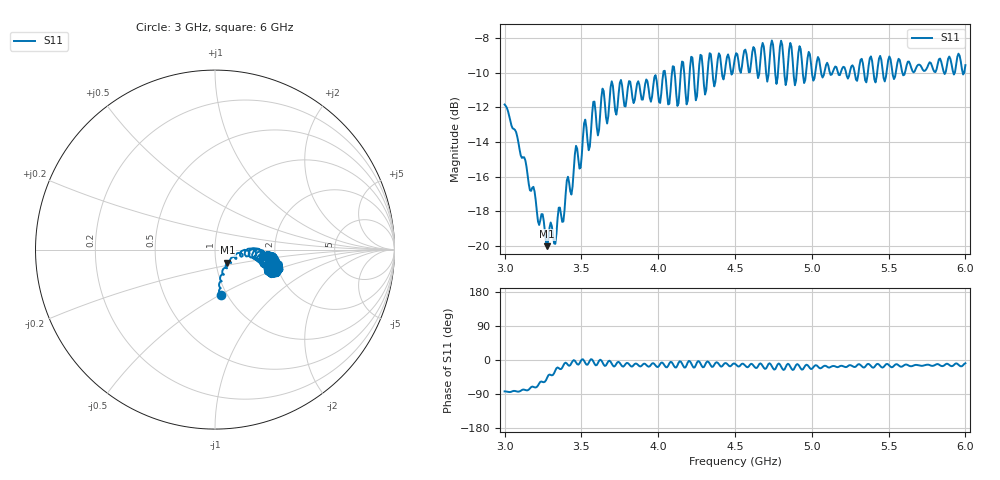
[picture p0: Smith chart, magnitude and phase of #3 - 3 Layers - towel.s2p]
!  02/07/2025  16:57:06
! Ref Plane: 0.000 mm
# MHZ S MA R  50
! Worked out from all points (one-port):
!   401 points, 3 GHz to 6 GHz, reference 50 ohm
!   lowest |S11| = -20.0 dB at 3.277 GHz (marker M1), VSWR 1.22, Z = 56.8 - j8.26 ohm
!   |S11| at or under -10 dB: start of sweep to 4.034 GHz; 4.044 GHz to 4.09 GHz (45.36 MHz wide, 1.12 % of centre); 4.107 GHz to 4.147 GHz (40.1 MHz wide, 0.972 % of centre)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
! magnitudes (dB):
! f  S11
! 3 GHz  -11.8
! 3.277 GHz  -20.0
! 3.375 GHz  -18.6
! 3.465 GHz  -14.2
! 3.555 GHz  -14.3
! 3.578 GHz  -11.7
! 3.607 GHz  -13.6
! 3.638 GHz  -10.9
! 3.667 GHz  -12.9
! 3.75 GHz  -10.6
! 4.013 GHz  -11.7
! 4.043 GHz  -9.9
! 4.065 GHz  -11.8
! 4.095 GHz  -9.6
! 4.125 GHz  -11.9
! 4.155 GHz  -9.3
! 4.185 GHz  -11.8
! 4.215 GHz  -9.1
! 4.245 GHz  -11.6
! 4.275 GHz  -9.0
! 4.305 GHz  -11.3
! 4.335 GHz  -8.9
! 4.365 GHz  -10.8
! 4.5 GHz  -9.1
! 4.875 GHz  -9.2
! 5.25 GHz  -9.9
! 5.625 GHz  -9.4
! 6 GHz  -9.6
